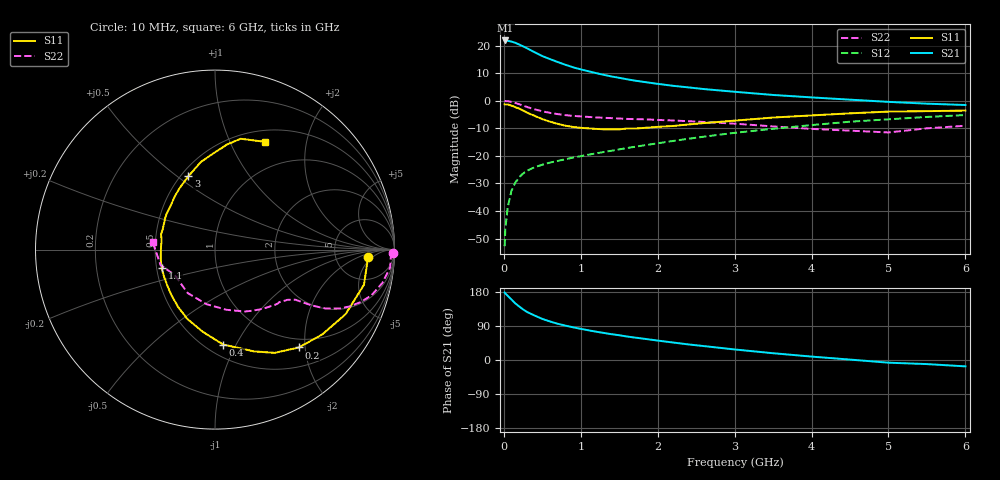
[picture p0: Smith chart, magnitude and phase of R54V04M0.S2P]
! SIEMENS Small Signal Semiconductors
! BFR183
! Si NPN RF Bipolar Junction Transistor in SOT23
! VCE = 4 V  IC = 4 mA
! Common Emitter S-Parameters:  May  1996
# GHz  S  MA  R  50
!  f  S11  S21  S12  S22
! GHz  MAG  ANG  MAG  ANG  MAG  ANG  MAG  ANG
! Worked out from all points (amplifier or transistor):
!   36 points, 10 MHz to 6 GHz, reference 50 ohm
!   highest |S21| = 21.8 dB at 20 MHz (marker M1)
!   |S21| within 3 dB of that: start of sweep to 312.4 MHz
!   unconditionally stable (mu >= 1): 1.161 GHz to 2.687 GHz
!   at 250 MHz: K = 0.36, MSG = 23.1 dB, |S12| = -26.4 dB
!   at 1.4 GHz: K = 1.06, MAG = 12.0 dB, |S12| = -18.2 dB
!   at 6 GHz: K = 0.88, MSG = 1.8 dB, |S12| = -5.2 dB
!   S11 on the Smith chart (normalised r, x): 10 MHz: 12, -4; 200 MHz: 0.83, -1.88; 400 MHz: 0.60, -0.89; 1.1 GHz: 0.53, -0.12; 3 GHz: 0.55, +0.55; 6 GHz: 0.64, +1.36
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0.01  0.8558 -2.8  12.26 178.0  0.0023 87.7  0.9925 -1.1
0.02  0.8511 -5.4  12.35 175.5  0.0048 89.8  0.9807 -2.3
0.05  0.8528 -13.3  12.18 169.5  0.0116 83.9  0.9808 -5.9
0.1  0.8118 -26.3  11.78 159.5  0.0235 76.6  0.9505 -11.3
0.15  0.7616 -38.4  11.19 149.2  0.0328 70.2  0.9082 -16.3
0.2  0.7179 -49.4  10.4 141.2  0.0408 66.2  0.8627 -19.8
0.25  0.6644 -60.0  9.659 133.5  0.0478 61.5  0.8142 -22.9
0.3  0.6069 -69.1  8.926 127.0  0.0535 59.1  0.7691 -25.2
0.4  0.5309 -85.1  7.554 117.3  0.0622 55.4  0.6952 -28.1
0.5  0.463 -98.5  6.437 108.5  0.0689 53.5  0.6413 -29.5
0.6  0.4154 -111.9  5.667 101.6  0.0755 52.7  0.6007 -30.4
0.7  0.3795 -122.9  5.02 95.7  0.0807 52.9  0.5702 -31.0
0.9  0.3338 -142.5  4.029 86.3  0.0928 53.5  0.5295 -31.9
1.1  0.3144 -160.6  3.41 78.4  0.1048 54.7  0.5071 -33.5
1.4  0.3013 176.2  2.745 68.1  0.1234 56.4  0.4826 -36.1
1.6  0.3123 164.4  2.444 62.0  0.1382 56.8  0.4672 -38.3
2.2  0.3474 135.5  1.859 46.1  0.186 56.6  0.4369 -47.1
3  0.4343 110.0  1.45 27.8  0.261 51.7  0.3827 -64.3
3.5  0.4943 99.2  1.269 17.9  0.3088 46.7  0.3413 -79.3
4.5  0.589 83.5  1.043 1.1  0.4155 35.2  0.2859 -122.2
5.5  0.6453 70.6  0.882 -10.8  0.5067 22.2  0.3152 -164.1
6  0.6612 65.2  0.834 -16.8  0.5491 13.9  0.3509 172.8
